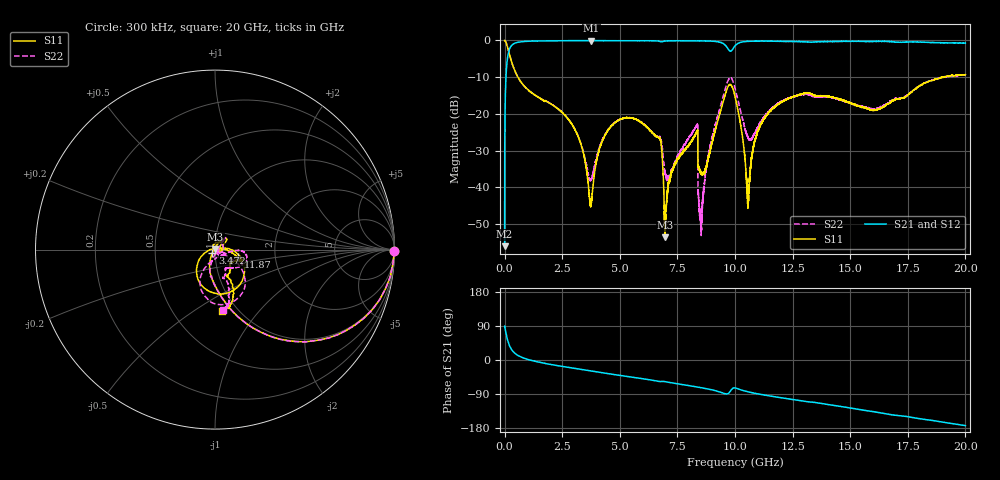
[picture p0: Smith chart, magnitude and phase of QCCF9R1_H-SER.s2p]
!{QCCF9R1}
!Johanson Technology Inc.
!www.johansontechnology.com
!Test Board Conditions:
!Substrate Type  RO4350B
!Substrate Thickness  10 mil
!Substrate Dk  3.66
!TL Type: GCPW
!TL Trace Width  21 mil
!TL Gap  20 mil
!Electrode orientation  Horizontal
!DUT TOPOLOGY	SERIES
!Mounting Pad LxW  16x21 mil
! Created Sat Jan  9 18:16:52 2021
# hz S ma R 50
! 2 Port Network Data from SP1.SP block
! freq  magS11  angS11  magS21  angS21  magS12  angS12  magS22  angS22
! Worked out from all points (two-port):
!   20001 points, 300 kHz to 20 GHz, reference 50 ohm
!   highest |S21| = -0.03 dB at 3.759 GHz (marker M1); lowest = -56.0 dB at 300 kHz (marker M2)
!   |S21| within 3 dB of the highest: 179.2 MHz to end of sweep
!   lowest |S11| = -53.6 dB at 6.965 GHz (marker M3), VSWR 1.00, Z = 50.2 + j0.146 ohm
!   |S11| at or under -10 dB: 581 MHz to 19.07 GHz (18.48 GHz wide, 188 % of centre); 19.07241 GHz to 19.0747 GHz (2.29 MHz wide, 0.012 % of centre); 19.07575 GHz to 19.07745 GHz (1.698 MHz wide, 0.0089 % of centre)
!   |S22| runs from -53.1 to 0.0 dB; largest |S21 - S12| = 0.015
!   S11 on the Smith chart (normalised r, x): 300 kHz: open; 3.472 GHz: 0.97, -0.04; 11.87 GHz: 1.29, -0.11; 20 GHz: 0.85, -0.65
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300000  0.999 -0.5  0.001584 88.9  0.001706 89.6  0.9986 -0.6
1.093e8  0.8498 -32.7  0.5233 57.0  0.5233 57.0  0.8495 -32.8
2.783e8  0.5423 -59.8  0.8344 29.7  0.8344 29.6  0.5414 -59.8
3.3343e9  0.03672 -122.7  0.9954 -25.1  0.9953 -25.0  0.03764 -97.8
3.4723e9  0.0243 -128.6  0.9951 -26.4  0.9951 -26.4  0.026 -89.4
3.7593e9  0.006394 128.9  0.9964 -29.1  0.9959 -29.1  0.01278 -16.1
4.1483e9  0.03568 64.3  0.9938 -32.7  0.994 -32.8  0.03729 40.7
4.7593e9  0.0749 51.1  0.992 -38.4  0.9914 -38.4  0.07549 48.6
6.6673e9  0.04787 23.2  0.9807 -56.2  0.981 -56.2  0.04834 26.4
6.9653e9  0.002098 44.0  0.982 -57.1  0.9817 -57.1  0.01587 -50.0
7.3263e9  0.01833 117.4  0.9908 -61.0  0.9909 -61.0  0.0187 -61.9
8.2863e9  0.05292 54.8  0.986 -70.5  0.9853 -70.5  0.06563 -27.5
8.5243e9  0.01617 -42.4  0.9869 -73.0  0.9865 -73.1  0.003516 28.8
9.2083e9  0.07133 4.4  0.9637 -82.0  0.9646 -81.9  0.08429 -29.4
9.7163e9  0.2411 -56.3  0.7524 -88.0  0.7527 -87.9  0.2927 -60.9
1.00003e10  0.1721 -126.1  0.8449 -73.8  0.844 -73.7  0.2235 -111.6
1.05653e10  0.006155 98.0  0.9733 -84.0  0.974 -83.9  0.04717 -81.0
1.09963e10  0.059 0.4  0.9805 -89.4  0.9799 -89.5  0.06609 -17.2
1.18693e10  0.1352 -18.5  0.975 -98.3  0.9763 -98.3  0.1391 -2.5
1.33343e10  0.1866 -29.8  0.9488 -111.2  0.9493 -111.3  0.1766 -24.8
1.66673e10  0.1367 -52.3  0.9681 -143.0  0.9593 -143.5  0.145 -66.8
2e10  0.3425 -83.8  0.9213 -173.2  0.913 -173.1  0.3411 -82.6
